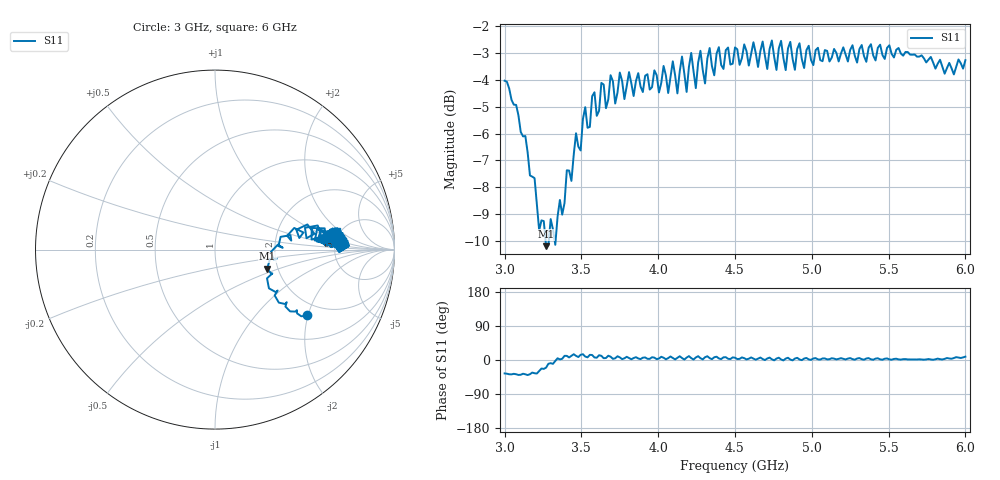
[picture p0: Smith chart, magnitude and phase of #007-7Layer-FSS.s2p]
!  05/08/2025  17:21:20
! Ref Plane: 0.000 mm
# MHZ S MA R  50
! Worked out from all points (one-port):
!   201 points, 3 GHz to 6 GHz, reference 50 ohm
!   lowest |S11| = -10.2 dB at 3.27 GHz (marker M1), VSWR 1.90, Z = 87.8 - j20.8 ohm
!   |S11| at or under -10 dB: 3.267 GHz to 3.287 GHz (20.35 MHz wide, 0.621 % of centre); 3.326464 GHz to 3.331896 GHz (5.432 MHz wide, 0.163 % of centre)
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3000  0.6284 -35.4
3270  0.3096 -20.2
3375  0.3543 3.1
3510  0.5336 15.2
3750  0.6508 7.0
4065  0.5961 4.9
4095  0.6829 5.5
4125  0.5952 5.8
4155  0.6968 5.2
4185  0.599 6.3
4215  0.7079 5.0
4245  0.6088 6.7
4275  0.7143 4.8
4305  0.621 7.3
4335  0.7227 4.9
4365  0.6431 7.3
4500  0.7246 6.1
4695  0.6988 -0.2
4725  0.7194 6.4
4755  0.696 -0.9
4785  0.7212 6.1
4815  0.6929 -1.1
4845  0.7215 5.9
4875  0.69 -0.9
4905  0.7197 5.8
5250  0.717 5.0
5625  0.7103 1.5
6000  0.6861 8.8
